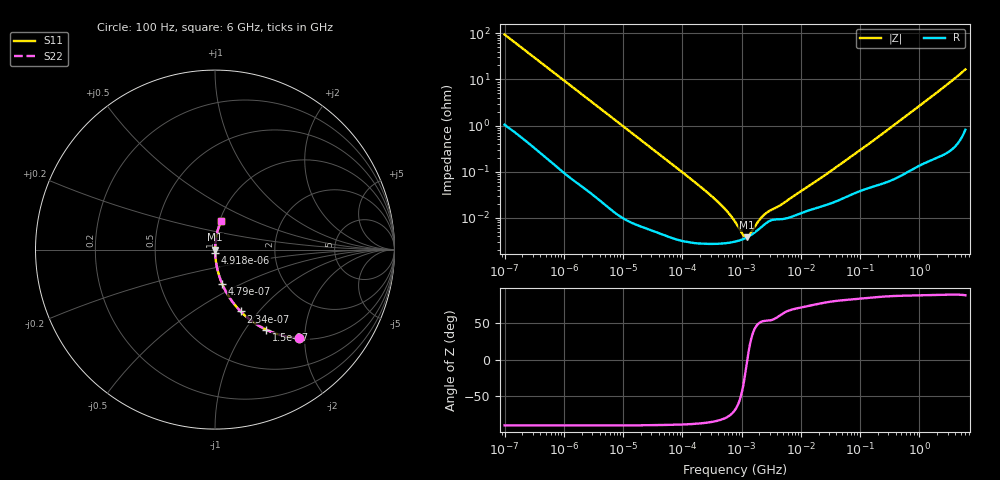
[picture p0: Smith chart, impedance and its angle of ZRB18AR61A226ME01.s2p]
!Murata Part Number: ZRB18AR61A226ME01
!These Parameters are Measured in Series Mode Connection
!Data Generated on Jun 10, 2025
!  o--ll--o
!Port1  Port2
!  o------o
!Operation Temp=25[degC], DC Bias Voltage=0[V]
!Freq. Start=100[Hz] Stop=6[GHz] 401[Steps]
# Hz S RI R 50
!Freq.(Hz) S11(Real) S11(Imag) S21(Real) S21(Imag) S12(Real) S12(Imag) S22(Real) S22(Imag)
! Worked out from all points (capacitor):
!   401 points, 100 Hz to 6 GHz, reference 50 ohm
!   read as one part in series: C = 16.9 uF near 109 Hz
!   lowest |Z| = 3.77 mohm at 1.212 MHz (marker M1)
!   series resonance near 1.251 MHz, so ESL is about 960 pH
!   S11 on the Smith chart (normalised r, x): 100 Hz: 1.02, -1.88; 150 Hz: 1.01, -1.26; 234 Hz: 1.01, -0.81; 479 Hz: 1.00, -0.40; 4.918 kHz: 1.00, -0.04; 6 GHz: 1.02, +0.33
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100  0.4693 -0.4935  0.5307 0.4935  0.5307 0.4935  0.4693 -0.4935
150  0.2863 -0.4464  0.7137 0.4464  0.7137 0.4464  0.2863 -0.4464
234  0.143 -0.3446  0.857 0.3446  0.857 0.3446  0.143 -0.3446
320  0.083 -0.2705  0.917 0.2705  0.917 0.2705  0.083 -0.2705
479  0.0397 -0.1901  0.9603 0.1901  0.9603 0.1901  0.0397 -0.1901
938  0.0112 -0.1005  0.9888 0.1005  0.9888 0.1005  0.0112 -0.1005
2008  0.00275 -0.0476  0.9973 0.0476  0.9973 0.0476  0.00275 -0.0476
4918  0.000577 -0.0196  0.9994 0.0196  0.9994 0.0196  0.000577 -0.0196
40335  5.24e-05 -0.00241  0.9999 0.00241  0.9999 0.00241  5.24e-05 -0.00241
241822  2.76e-05 -0.000391  1 0.000391  1 0.000391  2.76e-05 -0.000391
432798  2.77e-05 -0.000199  1 0.000199  1 0.000199  2.77e-05 -0.000199
677235  2.95e-05 -0.000102  1 0.000102  1 0.000102  2.95e-05 -0.000102
774597  3.06e-05 -7.75e-05  1 7.75e-05  1 7.75e-05  3.06e-05 -7.75e-05
1212075  3.74e-05 -4.8e-06  1 4.8e-06  1 4.8e-06  3.74e-05 -4.8e-06
1896632  5.51e-05 6.16e-05  0.9999 -6.16e-05  0.9999 -6.16e-05  5.51e-05 6.16e-05
2169299  6.38e-05 7.98e-05  0.9999 -7.98e-05  0.9999 -7.98e-05  6.38e-05 7.98e-05
2837864  8.31e-05 0.00011  0.9999 -0.00011  0.9999 -0.00011  8.31e-05 0.00011
4643984  9.36e-05 0.000168  0.9999 -0.000168  0.9999 -0.000168  9.36e-05 0.000168
1.555665e7  0.000154 0.000525  0.9998 -0.000525  0.9998 -0.000525  0.000154 0.000525
3.124326e8  0.000696 0.00857  0.9993 -0.00857  0.9993 -0.00857  0.000696 0.00857
1.873145e9  0.00432 0.0488  0.9957 -0.0488  0.9957 -0.0488  0.00432 0.0488
6e9  0.0338 0.1576  0.9662 -0.1576  0.9662 -0.1576  0.0338 0.1576
